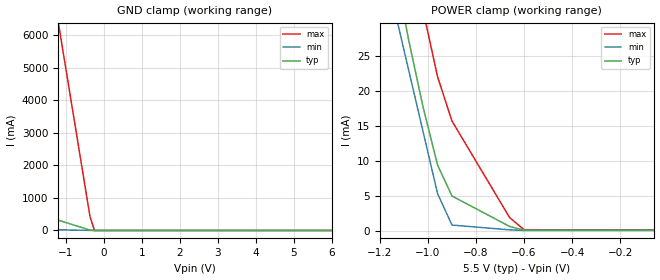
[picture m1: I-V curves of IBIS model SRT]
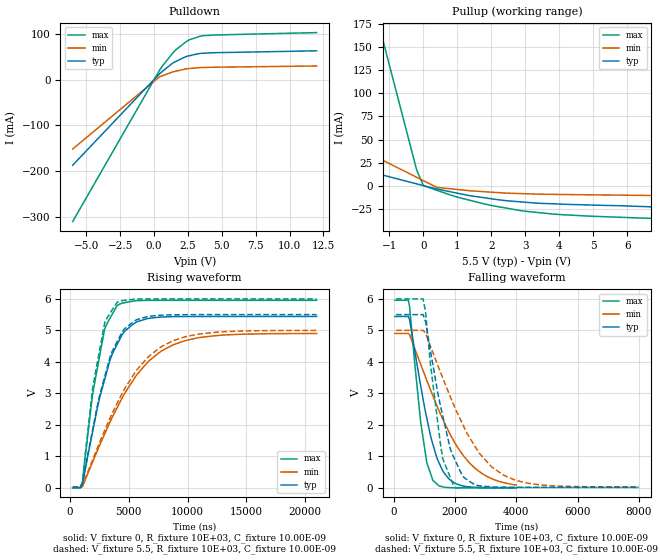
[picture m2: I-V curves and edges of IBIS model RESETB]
| IBIS file max821l.ibs created at Maxim Integrated Products
[IBIS ver]   3.2
[File name]   max821l.ibs
[File Rev]   1.0
[Date]   January 06, 2009
[Source]   Data was acquired from HSpice simulations.
[Notes]   This is a microprocessor voltage monitor.
[Disclaimer] Maxim Integrated Products hereby grants the user of this
   IBIS model a non-exclusive, nontransferable license to use
   this IBIS model under the following terms. Before using
   this IBIS model, the user should read this license. If the
   user does not accept these terms, the IBIS model should be
   returned to Maxim Integrated Products within 30 days.
   The user is granted this license only to use the IBIS model
   and is not granted rights to sell, load, rent, lease or
   license the IBIS model in whole or in part, or in modified
   form to anyone other than user. User may modify the IBIS
   model to suit its specific applications but rights to
   derivative works and such modifications shall belong to
   Maxim Integrated Products. This IBIS model is provided on
   an "AS IS" basis and Maxim Integrated Products makes
   absolutely no warranty with respect to the information
   contained herein.MAXIM INTEGRATED PRODUCTS DISCLAIMS AND
   CUSTOMER WAIVES ALL WARRANTIES, EXPRESS OR IMPLIED,
   INCLUDING WARRANTIES OF MERCHANTABILITY OR FITNESS FOR A
   PARTICULAR PURPOSE. The entire risk as to quality and
   performance is with the Customer. ACCORDINGLY, IN NO EVENT
   SHALL THE COMPANY BE LIABLE FOR ANY DAMAGES, WHETHER IN
   CONTRACT OR TORT,INCLUDING ANY LOST PROFITS OR OTHER
   INCIDENTAL, CONSEQUENTIAL, EXEMPLARY, OR PUNITIVE DAMAGES
   ARISING OUT OF THE USE OR APPLICATION OF THE IBIS model
   provided in this package.Further, Maxim Integrated Products
   reserves the right to make changes without notice to any
   product herein to improve reliability, function, or design.
   Maxim Integrated Products does not convey any license under
   patent rights or any other intellectual property rights,
   including those of third parties.
   Maxim Integrated Products is not obligated to provide
   maintenance or support for the licensed IBIS model.
[Copyright]   Copyright of Maxim Integrated Products.
|   Component MAX821L
[Component]   MAX821L
[Manufacturer]   Maxim Integrated Products
[Package]
|variable   typ   min   max
R_pkg   58.250E-03   53.000E-03   60.000E-03
L_pkg   1.043E-09   0.469E-09   1.307E-09
C_pkg   0.199E-12   0   0.200E-12
[Pin]  signal_name   model_name   R_pin   L_pin   C_pin
1   GND   GND   0.053   0.625n   0
2   /RESET\   RESETB   0.060   1.182n   0.200p
3   SRT   SRT   0.060   1.183n   0.200p
4   VCC   POWER   0.060   1.181n   0.199p
| Models and submodels in the file (2): SRT (Input), RESETB (Output)
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|   Set Reset Timeout Input
[Model]   SRT
|Signals   SRT
Model_type   Input
Vinl = 0.385V
Vinh = 4.950V
C_comp   4.339E-13   3.505E-13   5.274E-13
[Temperature Range]   25   -40   125
[Voltage Range]   5.50V   5.00V   6.00V
[Pullup Reference]   5.50V   5.00V   6.00V
[Pulldown Reference]   0.00V   0.00V   0.00V
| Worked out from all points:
|   GND clamp passes 1 mA (typ) near -0.25 V on its own axis
|   POWER clamp passes 1 mA (typ) near -0.68 V on its own axis
[POWER_clamp]
| Note that the [POWER_clamp] voltage table is referenced to Vcc
| and is calculated using Vtable=Vcc - Vmeasured.
|V(V)   I(typ)   I(min)   I(max)
-6V       992.8mA    986.6mA    1.003A
-1.14V    38.11mA    31.76mA    52.33mA
-1.08V    27.23mA    22.94mA    41.5mA
-1.02V    17.64mA    14.12mA    31.47mA
-960mV    9.399mA    5.302mA    22.04mA
-900mV    4.961mA    806.1uA    15.7mA
-660mV    605.3uA    117.1uA    1.872mA
-600mV    60.47uA    30.77uA    140.2uA
-60mV     55.01uA    27.8uA     100.3uA
[GND_clamp]
| Note that the [GND_clamp] voltage table is referenced to Gnd.
|V(V)   I(typ)   I(min)   I(max)
-5.88V    2.04A      123.6mA    39.99A
-1.2V     319.8mA    21.02mA    6.451A
-1.08V    275.7mA    18.39mA    5.591A
-360mV    11.03mA    2.626mA    430.3mA
-240mV    2.554uA    1.319uA    16.86uA
6V        -59.37uA   -32.97uA   -99.28uA
|   Reset Output
[Model]   RESETB
|Signals   RESETB
Model_type   Output
Polarity   Inverting
Vmeas = 2.75V
C_comp   6.106E-13   4.933E-13   7.407E-13
[Temperature Range]   25   125   -40
[Voltage Range]   5.50V   5.00V   6.00V
[Pullup Reference]   5.50V   5.00V   6.00V
[Pulldown Reference]   0.00V   0.00V   0.00V
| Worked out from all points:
|   slope of the pulldown table from 0 to 0.825 V, typ, clamps not added: 36.1 ohm
|   slope of the pullup table from 0 to 0.825 V, typ, clamps not added: 120 ohm
|   rising waveform, V_fixture 0, R_fixture 10E+03, C_fixture 10.00E-09: 20-80 % time 2.18us typ, 4.35us min, 1.45us max; typ from 0 V to 5.44 V
|   falling waveform, V_fixture 0, R_fixture 10E+03, C_fixture 10.00E-09: 20-80 % time 681ns typ, 1.38us min, 408ns max; typ from 5.44 V to 0 V
|   rising waveform, V_fixture 5.5, R_fixture 10E+03, C_fixture 10.00E-09: 20-80 % time 2.14us typ, 4.24us min, 1.39us max; typ from 0.016 V to 5.5 V
|   falling waveform, V_fixture 5.5, R_fixture 10E+03, C_fixture 10.00E-09: 20-80 % time 705ns typ, 1.47us min, 443ns max; typ from 5.5 V to 0.016 V
[Pullup]
| Note that the [Pullup] voltage table is referenced to Vcc
| and is calculated using Vtable=Vcc - Vmeasured.
|V(V)   I(typ)   I(min)   I(max)
-6V       57.19mA    115.9mA    836.6mA
-1.4V     13.45mA    31.28mA    186.7mA
-1.2V     11.54mA    27.6mA     158.4mA
-200mV    2.035mA    9.201mA    17.1mA
0V        134.2uA    5.524mA    92.42uA
400mV     -3.568mA   -1.831mA   -4.993mA
800mV     -6.571mA   -3.3mA     -10.08mA
1.4V      -10.96mA   -5.504mA   -16.02mA
2V        -14.08mA   -6.952mA   -21.34mA
3V        -17.84mA   -8.641mA   -27.6mA
4V        -19.79mA   -9.405mA   -31.14mA
12V       -29.69mA   -12.65mA   -42.19mA
[Pulldown]
| Note that the [Pulldown] voltage table is referenced to Gnd.
|V(V)   I(typ)   I(min)   I(max)
-6V       -187.4mA   -151.9mA   -310.5mA
400mV     12.35mA    5.844mA    19.78mA
600mV     17.22mA    8.06mA     28.83mA
1.4V      36.2mA     16.92mA    58.54mA
1.6V      39.17mA    18.24mA    64.75mA
2.4V      50.66mA    23.51mA    83.29mA
2.6V      52.01mA    24.05mA    86.76mA
3.6V      57.46mA    26.38mA    95.9mA
12V       62.82mA    29.64mA    102.7mA
[Ramp]
|variable   typ   min   max
dV/dt_r   3.265/2.240E-06   2.941/4.516E-06   3.572/1.464E-06
dV/dt_f   3.265/7.057E-07   2.941/1.488E-06   3.572/4.380E-07
R_load = 10E+03
[Rising Waveform]
V_fixture = 0
V_fixture_min = 0
V_fixture_max = 0
R_fixture = 10E+03
L_fixture = 0
C_fixture = 10.00E-09
|Time   V(typ)   V(min)   V(max)
210ns     0V         0V         0V
1.05us    97.58mV    38.66mV    171.1mV
1.89us    1.74V      801.8mV    2.916V
2.94us    3.443V     1.712V     5.048V
3.99us    4.546V     2.536V     5.784V
4.62us    4.965V     2.987V     5.879V
5.67us    5.27V      3.589V     5.944V
8.82us    5.436V     4.549V     5.954V
13us      5.442V     4.85V      5.954V
21us      5.442V     4.901V     5.954V
[Falling Waveform]
V_fixture = 0
V_fixture_min = 0
V_fixture_max = 0
R_fixture = 10E+03
L_fixture = 0
C_fixture = 10.00E-09
|Time   V(typ)   V(min)   V(max)
40ns      5.442V     4.902V     5.956V
480ns     5.442V     4.902V     5.956V
520ns     5.34V      4.865V     5.76V
880ns     3.255V     3.928V     2.104V
1.08us    2.217V     3.417V     809.4mV
1.28us    1.382V     2.92V      240.6mV
1.44us    879.3mV    2.542V     97.11mV
1.8us     287.6mV    1.781V     8.093mV
2.48us    28.7mV     785.1mV    51.29uV
4us       131.5uV    89.6mV     0V
[Rising Waveform]
V_fixture = 5.5
V_fixture_min = 5.0
V_fixture_max = 6.0
R_fixture = 10E+03
L_fixture = 0
C_fixture = 10.00E-09
|Time   V(typ)   V(min)   V(max)
210ns     16.34mV    30.33mV    10.83mV
1.05us    116.4mV    70.88mV    193.7mV
1.89us    1.796V     869.7mV    3.102V
2.94us    3.528V     1.82V      5.242V
3.99us    4.632V     2.673V     5.889V
4.62us    5.046V     3.135V     5.954V
5.67us    5.34V      3.742V     5.995V
8.82us    5.494V     4.678V     6V
12.8us    5.499V     4.95V      6V
21us      5.5V       4.999V     6V
[Falling Waveform]
V_fixture = 5.5
V_fixture_min = 5.0
V_fixture_max = 6.0
R_fixture = 10E+03
L_fixture = 0
C_fixture = 10.00E-09
|Time   V(typ)   V(min)   V(max)
80ns      5.5V       5V         6V
960ns     5.5V       5V         6V
1.04us    5.281V     4.912V     5.589V
1.2us     4.361V     4.5V       3.934V
1.6us     2.295V     3.489V     927.1mV
2us       888.5mV    2.537V     1.429mV
2.24us    386.2mV    2.043V     7.569mV
2.64us    101.7mV    1.34V      11.16mV
3.6us     18.89mV    394.9mV    10.83mV
8us       16.34mV    30.78mV    10.83mV
